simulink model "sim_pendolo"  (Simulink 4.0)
settings: Solver=ode45  StartTime=0.0  StopTime=10.0  RelTol=1e-3
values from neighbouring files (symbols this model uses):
  csi = 0.05    [Pendolo.m]    (also in PendoloPoincare.m; pendolo_param.m)
  g = 9.81    [Pendolo.m]    (also in PendoloPoincare.m; pendolo_param.m)
  L = 0.1    [Pendolo.m]    (also in PendoloPoincare.m; pendolo_param.m)
  lamda = 0.1    [Pendolo.m]    (also in PendoloPoincare.m = 1; pendolo_param.m)
  r = 1.8    [Pendolo.m]    (also in PendoloPoincare.m = 1.4; pendolo_param.m = 1.25)
  x0 = pi    (= 3.14159265359)    [Pendolo.m]    (also in PendoloPoincare.m = 1.57079632679; pendolo_param.m)
  xp0 = 0.01    [Pendolo.m]    (also in PendoloPoincare.m = 0; pendolo_param.m = 0)

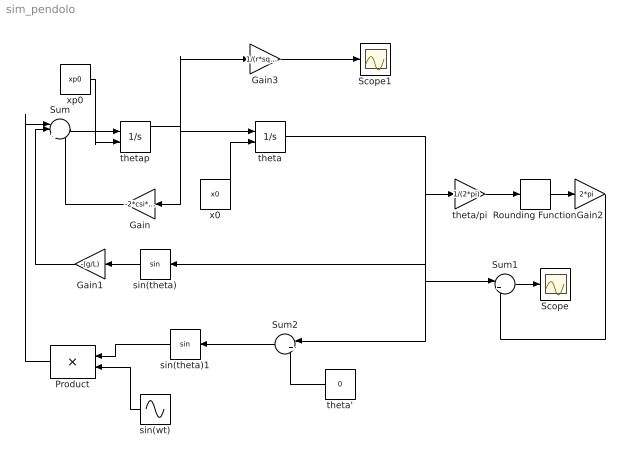
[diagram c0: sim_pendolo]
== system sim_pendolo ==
  Gain : Gain  Orientation=left  Gain=-2*csi*sqrt(g/L)  Multiplication=Element-wise(K.*u)  SaturateOnIntegerOverflow=on
  Gain1 : Gain  Orientation=left  Gain=-(g/L)  Multiplication=Element-wise(K.*u)  SaturateOnIntegerOverflow=on
  Gain2 : Gain  Gain=2*pi  Multiplication=Element-wise(K.*u)  SaturateOnIntegerOverflow=on
  Gain3 : Gain  Gain=1/(r*sqrt(g/L))  Multiplication=Element-wise(K.*u)  SaturateOnIntegerOverflow=on
  Product : Product  Orientation=left  Inputs=2  Multiplication=Element-wise(.*)  SaturateOnIntegerOverflow=on
  Rounding Function : Rounding  Operator=round
  Scope : Scope
  Scope1 : Scope
  Sum : Sum  Inputs=|+++  SaturateOnIntegerOverflow=on
  Sum1 : Sum  Inputs=|+-  SaturateOnIntegerOverflow=on
  Sum2 : Sum  Orientation=left  Inputs=|++  SaturateOnIntegerOverflow=on
  sin(theta) : Trigonometry  Orientation=left  Operator=sin  OutputSignalType=auto
  sin(theta)1 : Trigonometry  Orientation=left  Operator=sin  OutputSignalType=auto
  sin(wt) : Sin  Orientation=left  SineType=Time-based  Amplitude=(g/L)*lamda*r^2  Bias=0  Frequency=r*sqrt(g/L)  Phase=0  Samples=10  SampleTime=0
  theta : Integrator  ExternalReset=none  InitialConditionSource=external  InitialCondition=0  LimitOutput=off  UpperSaturationLimit=inf  LowerSaturationLimit=-inf  ShowSaturationPort=off  ShowStatePort=off  AbsoluteTolerance=auto
  theta' : Constant  Orientation=left  Value=0
  theta/pi : Gain  Gain=1/(2*pi)  Multiplication=Element-wise(K.*u)  SaturateOnIntegerOverflow=on
  thetap : Integrator  ExternalReset=none  InitialConditionSource=external  InitialCondition=0  LimitOutput=off  UpperSaturationLimit=inf  LowerSaturationLimit=-inf  ShowSaturationPort=off  ShowStatePort=off  AbsoluteTolerance=auto
  x0 : Constant  Value=x0
  xp0 : Constant  Value=xp0
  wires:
  thetap/1 -> theta/1, Gain/1, Gain3/1
  Gain/1 -> Sum/3
  Sum/1 -> thetap/1
  theta/1 -> sin(theta)/1, Sum1/1, Sum2/1, theta/pi/1
  sin(theta)/1 -> Gain1/1
  Gain1/1 -> Sum/2
  sin(wt)/1 -> Product/2
  Product/1 -> Sum/1
  theta/pi/1 -> Rounding Function/1
  Rounding Function/1 -> Gain2/1
  Gain2/1 -> Sum1/2
  Gain3/1 -> Scope1/1
  xp0/1 -> thetap/2
  x0/1 -> theta/2
  Sum1/1 -> Scope/1
  sin(theta)1/1 -> Product/1
  Sum2/1 -> sin(theta)1/1
  theta'/1 -> Sum2/2
